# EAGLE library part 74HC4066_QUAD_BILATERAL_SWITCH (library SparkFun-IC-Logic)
Nexperia Quad Bilateral Switch The 74HC4066 is a quad single pole, single throw analog switch. Each switch features two input/output terminals (nY and nZ) and an active HIGH enable input (nE). When nE is LOW, the analog switch is turned off. Inputs include clamp diodes. This enables the use of current limiting resistors to interface inputs to voltages in excess of VCC. Datasheet
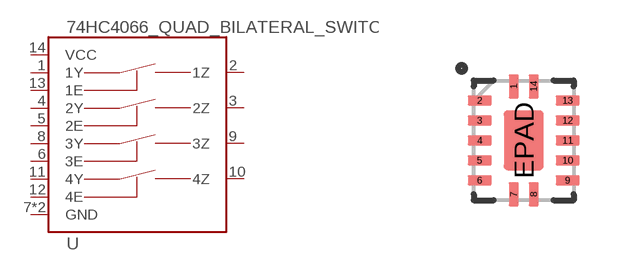
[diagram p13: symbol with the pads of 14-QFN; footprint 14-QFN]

Designator prefix -

## 74HC4066_QUAD_BILATERAL_SWITCH_QFN (PROD_ID: IC-16528)  [14-QFN]
1  1Y
2  1Z
3  2Z
4  2Y
5  2E
6  3E
7  GND
8  3Y
9  3Z
10  4Z
11  4Y
12  4E
13  1E
14  VCC
EPAD  GND

## Footprint 14-QFN (pad centres in mm)
36-QFN
smd 0.25 x 0.6: 1 -0.25,1.35; 7 -0.25,-1.35; 8 0.25,-1.35; 14 0.25,1.35
smd 0.6 x 0.25: 2 -1.1,1; 3 -1.1,0.5; 4 -1.1,0; 5 -1.1,-0.5; 6 -1.1,-1; 9 1.1,-1; 10 1.1,-0.5; 11 1.1,0; 12 1.1,0.5; 13 1.1,1
smd 1 x 1.5: EPAD 0,0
